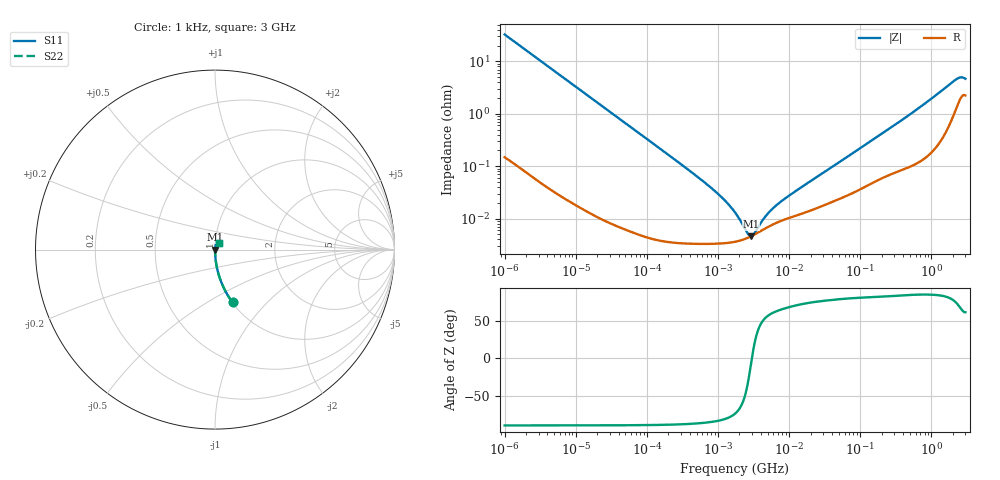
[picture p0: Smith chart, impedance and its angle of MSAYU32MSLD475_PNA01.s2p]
! MSAYU32MSLD475_PNA01  S-PARAMETER MODEL  ( Standard Model )
! Model Generated by TAIYO YUDEN Corporation (http://www.ty-top.com)
! Version 1.0
! TAIYO YUDEN Control No. 220601
! Copyright(c) 2014 TAIYO YUDEN CO.,LTD. All Rights Reserved.
! Product Description (link to TY-COMPAS)
! https://ds.yuden.co.jp/TYCOMPAS/or/detail?pn=MSAYU32MSLD475KPNA01&u=M
! Products Name : Multilayer Ceramic Capacitors
! Characteristics :
!  Capacitance : 4.7 [uF] , Rated Voltage : 50 [V] , TCC : X5R
!  Case Size : 3.2 x 2.5 / 0.126 x 0.098 [mm/inch] , Thickness : 2.5 / 0.098 [mm/inch]
!  (Conditions: Temperature = 25 [degC] , DC Bias Voltage = 0 [V])
! External Node Assignments :
!  1  o---| |---o  2
! GND o---------o GND
! Frequency Range : 1kHz  -  3GHz  [ 401 STEP ]
# MHZ S RI R 50
! Freq[MHz].  S11 Real  S11 Imag  S21 Real  S21 Imag  S12 Real  S12 Imag  S22 Real  S22 Imag
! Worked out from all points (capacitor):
!   401 points, 1 kHz to 3 GHz, reference 50 ohm
!   read as one part in series: C = 4.86 uF near 1.077 kHz
!   lowest |Z| = 4.63 mohm at 2.919 MHz (marker M1)
!   series resonance near 2.994 MHz, so ESL is about 580 pH
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0.001  0.0976 -0.2945  0.9024 0.2945  0.9024 0.2945  0.0976 -0.2945
0.001624  0.0399 -0.1934  0.9601 0.1934  0.9601 0.1934  0.0399 -0.1934
0.002948  0.0127 -0.1098  0.9873 0.1098  0.9873 0.1098  0.0127 -0.1098
0.005557  0.00377 -0.0589  0.9962 0.0589  0.9962 0.0589  0.00377 -0.0589
0.01216  0.000887 -0.027  0.9991 0.027  0.9991 0.027  0.000887 -0.027
0.147855  4.32e-05 -0.00224  1 0.00224  1 0.00224  4.32e-05 -0.00224
0.821683  3.31e-05 -0.000373  1 0.000373  1 0.000373  3.31e-05 -0.000373
1.285341  3.41e-05 -0.00021  1 0.00021  1 0.00021  3.41e-05 -0.00021
1.732051  3.61e-05 -0.000126  1 0.000126  1 0.000126  3.61e-05 -0.000126
1.937042  3.73e-05 -9.83e-05  1 9.83e-05  1 9.83e-05  3.73e-05 -9.83e-05
2.087011  3.84e-05 -8.04e-05  1 8.04e-05  1 8.04e-05  3.84e-05 -8.04e-05
2.919173  4.6e-05 -5.3e-06  1 5.3e-06  1 5.3e-06  4.6e-05 -5.3e-06
4.083148  5.9e-05 6.35e-05  0.9999 -6.35e-05  0.9999 -6.35e-05  5.9e-05 6.35e-05
4.399271  6.25e-05 7.83e-05  0.9999 -7.83e-05  0.9999 -7.83e-05  6.25e-05 7.83e-05
5.928204  7.74e-05 0.000137  0.9999 -0.000137  0.9999 -0.000137  7.74e-05 0.000137
7.696136  9.04e-05 0.000192  0.9999 -0.000192  0.9999 -0.000192  9.04e-05 0.000192
21.06097  0.000146 0.000525  0.9999 -0.000525  0.9999 -0.000525  0.000146 0.000525
256.0921  0.000706 0.00516  0.9993 -0.00516  0.9993 -0.00516  0.000706 0.00516
727.4359  0.00148 0.014  0.9985 -0.014  0.9985 -0.014  0.00148 0.014
2144.796  0.0127 0.0416  0.9873 -0.0416  0.9873 -0.0416  0.0127 0.0416
2489.759  0.0198 0.044  0.9802 -0.044  0.9802 -0.044  0.0198 0.044
3000  0.0235 0.039  0.9765 -0.039  0.9765 -0.039  0.0235 0.039
